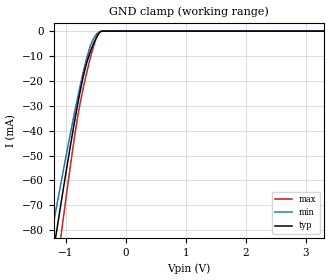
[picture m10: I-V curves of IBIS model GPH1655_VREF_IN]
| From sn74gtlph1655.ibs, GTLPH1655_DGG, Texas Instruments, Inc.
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[Model]   GPH1655_VREF_IN
Model_type  Input
Vinl=0.8
Vinh=2.0
| variable   typ   min   max
C_comp   19.00pF   14.09pF   22.74pF
[Temperature Range]   40   100   -40
| Ambient temperature   25   85   -40
[Voltage range]   3.3   3.15   3.45
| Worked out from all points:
|   GND clamp passes 1 mA (typ) near -0.45 V on its own axis
[GND Clamp]
| GPH1655_VREF_IN
|   Voltage   I(typ)   I(min)   I(max)
-5.5V     -820.7mA   -702.8mA   -996.7mA
-1.265V   -97.69mA   -85.25mA   -116.9mA
-1.215V   -89.89mA   -78.6mA    -107.4mA
-1.17V    -82.93mA   -72.65mA   -98.92mA
-1.125V   -76.03mA   -66.75mA   -90.52mA
-1.085V   -69.95mA   -61.56mA   -83.13mA
-1.045V   -63.93mA   -56.41mA   -75.82mA
-815mV    -31.08mA   -28.13mA   -36.3mA
-705mV    -17.79mA   -16.04mA   -22.42mA
-570mV    -6.995mA   -4.687mA   -8.829mA
-430mV    -397.5uA   -211.4uA   -298.5uA
3.3V      1.471nA    4.967nA    7.249nA
